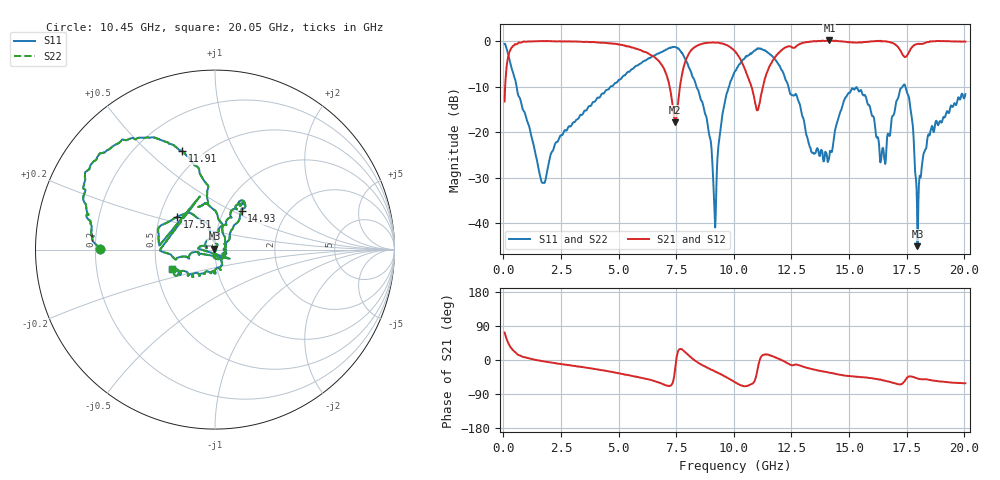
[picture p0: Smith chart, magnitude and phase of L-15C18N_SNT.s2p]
#	mhz	s	ma	r	50
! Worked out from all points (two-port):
!   1001 points, 50 MHz to 20.05 GHz, reference 50 ohm
!   highest |S21| = 0.22 dB at 14.15 GHz (marker M1); lowest = -17.8 dB at 7.45 GHz (marker M2)
!   |S21| within 3 dB of the highest: 233.5 MHz to 6.329 GHz (6.095 GHz wide, 186 % of centre); 11.9 GHz to 17.31 GHz (5.419 GHz wide, 37.1 % of centre)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
!   lowest |S11| = -45.0 dB at 17.97 GHz (marker M3), VSWR 1.01, Z = 49.7 + j0.453 ohm
!   |S11| at or under -10 dB: 571.5 MHz to 4.632 GHz (4.06 GHz wide, 156 % of centre); 12.37 GHz to 17.31 GHz (4.943 GHz wide, 33.3 % of centre); 17.45 GHz to end of sweep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
!   |S22| runs from -45.0 to -0.5 dB; largest |S21 - S12| = 0
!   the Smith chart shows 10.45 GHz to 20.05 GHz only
!   S11 on the Smith chart (normalised r, x): 10.45 GHz: 0.22, +0.00; 11.91 GHz: 0.39, +0.65; 14.93 GHz: 1.21, +0.56; 17.51 GHz: 0.62, +0.24; 20.05 GHz: 0.60, -0.14
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50  0.9402 166.9  0.2188 72.5  0.2188 72.5  0.9402 166.9
570  0.318 108.6  0.9329 16.9  0.9329 16.9  0.318 108.6
1710  0.02787 -0.1  1.008 -3.1  1.008 -3.1  0.02787 -0.1
3390  0.1553 -96.4  0.9927 -18.4  0.9927 -18.4  0.1553 -96.4
6730  0.7359 -151.3  0.6123 -59.3  0.6123 -59.3  0.7359 -151.3
7450  0.8691 166.0  0.129 -24.6  0.129 -24.6  0.8691 166.0
7890  0.6431 123.1  0.5984 20.9  0.5984 20.9  0.6431 123.1
8730  0.1693 69.1  0.955 -16.7  0.955 -16.7  0.1693 69.1
9170  0.01146 2.4  0.9698 -29.8  0.9698 -29.8  0.01146 2.4
9550  0.1804 -135.4  0.9431 -41.1  0.9431 -41.1  0.1804 -135.4
10050  0.472 -156.3  0.7812 -58.4  0.7812 -58.4  0.472 -156.3
10450  0.6427 179.9  0.5183 -69.1  0.5183 -69.1  0.6427 179.9
11030  0.8424 149.2  0.1759 -23.7  0.1759 -23.7  0.8424 149.2
11910  0.5765 108.3  0.7351 4.2  0.7351 4.2  0.5765 108.3
13390  0.05984 13.9  0.9984 -24.0  0.9984 -24.0  0.05984 13.9
14150  0.05509 10.7  1.026 -33.5  1.026 -33.5  0.05509 10.7
14930  0.2608 55.1  0.985 -42.1  0.985 -42.1  0.2608 55.1
16730  0.09213 -161.9  0.9901 -56.9  0.9901 -56.9  0.09213 -161.9
17510  0.278 138.8  0.6926 -47.2  0.6926 -47.2  0.278 138.8
17970  0.0056 125.4  0.9423 -48.5  0.9423 -48.5  0.0056 125.4
18510  0.09531 -68.8  0.9979 -52.7  0.9979 -52.7  0.09531 -68.8
20050  0.2629 -155.1  0.9952 -61.4  0.9952 -61.4  0.2629 -155.1
